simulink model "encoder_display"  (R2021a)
settings: Solver=FixedStepDiscrete  StartTime=0.0  StopTime=Inf  RelTol=1e-3  EnableMultiTasking=on
undefined symbols (not defined in the file or in its folder): Count, edge, falling, resolution, rising, the
libraries: c2806xlib x10, simulink x1, c280xlib x1

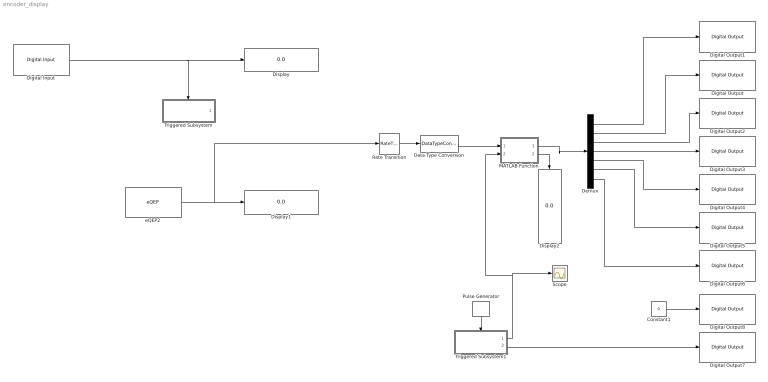
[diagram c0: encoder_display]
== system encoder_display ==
  Constant1 : Constant  Value=0
  Data Type Conversion : DataTypeConversion  OutDataTypeStr=uint16
  Demux : Demux  Outputs=7
  Digital Input : c2806xlib/Digital Input  Commented=on  GPIO_Number=GPIO50~GPIO55  GPIO_Bit0=off  GPIO_Bit1=off  GPIO_Bit2=off  GPIO_Bit3=off  GPIO_Bit4=on  GPIO_Bit5=off  GPIO_Bit6=off  GPIO_Bit7=off  sampleTime=0.1  dataType=auto  GPIO_Bit0_Qualification=Sync to SYSCLKOUT  GPIO_Bit1_Qualification=Sync to SYSCLKOUT  GPIO_Bit2_Qualification=Sync to SYSCLKOUT  GPIO_Bit3_Qualification=Sync to SYSCLKOUT  GPIO_Bit4_Qualification=Sync to SYSCLKOUT  GPIO_Bit5_Qualification=Sync to SYSCLKOUT  GPIO_Bit6_Qualification=Sync to SYSCLKOUT  GPIO_Bit7_Qualification=Sync to SYSCLKOUT  Qualification_Period=-1
  Digital Output : c2806xlib/Digital Output  GPIO_Number=GPIO16~GPIO23  GPIO_Bit0=off  GPIO_BIT0_Toggle=off  GPIO_Bit1=off  GPIO_BIT1_Toggle=off  GPIO_Bit2=off  GPIO_BIT2_Toggle=off  GPIO_Bit3=on  GPIO_BIT3_Toggle=off  GPIO_Bit4=off  GPIO_BIT4_Toggle=off  GPIO_Bit5=off  GPIO_BIT5_Toggle=off  GPIO_Bit6=off  GPIO_BIT6_Toggle=off  GPIO_Bit7=off  GPIO_BIT7_Toggle=off
  Digital Output1 : c2806xlib/Digital Output  GPIO_Number=GPIO50~GPIO55  GPIO_Bit0=off  GPIO_BIT0_Toggle=off  GPIO_Bit1=off  GPIO_BIT1_Toggle=off  GPIO_Bit2=on  GPIO_BIT2_Toggle=off  GPIO_Bit3=off  GPIO_BIT3_Toggle=off  GPIO_Bit4=off  GPIO_BIT4_Toggle=off  GPIO_Bit5=off  GPIO_BIT5_Toggle=off  GPIO_Bit6=off  GPIO_BIT6_Toggle=off  GPIO_Bit7=off  GPIO_BIT7_Toggle=off
  Digital Output2 : c2806xlib/Digital Output  GPIO_Number=GPIO8~GPIO15  GPIO_Bit0=off  GPIO_BIT0_Toggle=off  GPIO_Bit1=off  GPIO_BIT1_Toggle=off  GPIO_Bit2=off  GPIO_BIT2_Toggle=off  GPIO_Bit3=off  GPIO_BIT3_Toggle=off  GPIO_Bit4=off  GPIO_BIT4_Toggle=off  GPIO_Bit5=on  GPIO_BIT5_Toggle=off  GPIO_Bit6=off  GPIO_BIT6_Toggle=off  GPIO_Bit7=off  GPIO_BIT7_Toggle=off
  Digital Output3 : c2806xlib/Digital Output  GPIO_Number=GPIO0~GPIO7  GPIO_Bit0=off  GPIO_BIT0_Toggle=off  GPIO_Bit1=off  GPIO_BIT1_Toggle=off  GPIO_Bit2=off  GPIO_BIT2_Toggle=off  GPIO_Bit3=off  GPIO_BIT3_Toggle=off  GPIO_Bit4=off  GPIO_BIT4_Toggle=off  GPIO_Bit5=on  GPIO_BIT5_Toggle=off  GPIO_Bit6=off  GPIO_BIT6_Toggle=off  GPIO_Bit7=off  GPIO_BIT7_Toggle=off
  Digital Output4 : c2806xlib/Digital Output  GPIO_Number=GPIO16~GPIO23  GPIO_Bit0=off  GPIO_BIT0_Toggle=off  GPIO_Bit1=on  GPIO_BIT1_Toggle=off  GPIO_Bit2=off  GPIO_BIT2_Toggle=off  GPIO_Bit3=off  GPIO_BIT3_Toggle=off  GPIO_Bit4=off  GPIO_BIT4_Toggle=off  GPIO_Bit5=off  GPIO_BIT5_Toggle=off  GPIO_Bit6=off  GPIO_BIT6_Toggle=off  GPIO_Bit7=off  GPIO_BIT7_Toggle=off
  Digital Output5 : c2806xlib/Digital Output  GPIO_Number=GPIO0~GPIO7  GPIO_Bit0=off  GPIO_BIT0_Toggle=off  GPIO_Bit1=off  GPIO_BIT1_Toggle=off  GPIO_Bit2=off  GPIO_BIT2_Toggle=off  GPIO_Bit3=off  GPIO_BIT3_Toggle=off  GPIO_Bit4=on  GPIO_BIT4_Toggle=off  GPIO_Bit5=off  GPIO_BIT5_Toggle=off  GPIO_Bit6=off  GPIO_BIT6_Toggle=off  GPIO_Bit7=off  GPIO_BIT7_Toggle=off
  Digital Output6 : c2806xlib/Digital Output  GPIO_Number=GPIO40~GPIO44  GPIO_Bit0=off  GPIO_BIT0_Toggle=off  GPIO_Bit1=off  GPIO_BIT1_Toggle=off  GPIO_Bit2=off  GPIO_BIT2_Toggle=off  GPIO_Bit3=off  GPIO_BIT3_Toggle=off  GPIO_Bit4=on  GPIO_BIT4_Toggle=off  GPIO_Bit5=off  GPIO_BIT5_Toggle=off  GPIO_Bit6=off  GPIO_BIT6_Toggle=off  GPIO_Bit7=off  GPIO_BIT7_Toggle=off
  Digital Output7 : c2806xlib/Digital Output  GPIO_Number=GPIO0~GPIO7  GPIO_Bit0=on  GPIO_BIT0_Toggle=off  GPIO_Bit1=on  GPIO_BIT1_Toggle=off  GPIO_Bit2=on  GPIO_BIT2_Toggle=off  GPIO_Bit3=on  GPIO_BIT3_Toggle=off  GPIO_Bit4=off  GPIO_BIT4_Toggle=off  GPIO_Bit5=off  GPIO_BIT5_Toggle=off  GPIO_Bit6=off  GPIO_BIT6_Toggle=off  GPIO_Bit7=off  GPIO_BIT7_Toggle=off
  Digital Output8 : c2806xlib/Digital Output  GPIO_Number=GPIO16~GPIO23  GPIO_Bit0=on  GPIO_BIT0_Toggle=off  GPIO_Bit1=off  GPIO_BIT1_Toggle=off  GPIO_Bit2=off  GPIO_BIT2_Toggle=off  GPIO_Bit3=off  GPIO_BIT3_Toggle=off  GPIO_Bit4=off  GPIO_BIT4_Toggle=off  GPIO_Bit5=off  GPIO_BIT5_Toggle=off  GPIO_Bit6=off  GPIO_BIT6_Toggle=off  GPIO_Bit7=off  GPIO_BIT7_Toggle=off
  Display : Display
  Display1 : Display
  Display2 : Display
  MATLAB Function : MATLAB Function  TreatAsAtomicUnit=on
  Pulse Generator : DiscretePulseGenerator  SampleTime=0.0005
  Rate Transition : RateTransition
  Scope : Scope
  Triggered Subsystem : Subsystem  Commented=on  TreatAsAtomicUnit=on
  Triggered Subsystem1 : Subsystem  TreatAsAtomicUnit=on
  eQEP2 : c280xlib/eQEP  useModule=eQEP2  pcInputmode=Quadrature-count  externalClockrate=2x resolution: Count the rising/falling edge  swapPolarityselection=Clockwise  qdfOutputport=off  qapPolarityselection=off  qbpPolarityselection=off  qipPolarityselection=off  qspPolarityselection=off  igatePolarityselection=off  sampleTime=0.01  pcOutputport=on  pcMaximumvalue=999  indexInitializationcheck=off  indexInitializationevent=Rising edge  strobeInitializationcheck=off  strobeInitializationevent=Rising edge  softwareInitializationcheck=on  softwareInitializationsource=Set to init value at start up  softwareInitializationmode=on  pcInitialvalue=0  pcResetmode=Reset on an index event  ieloutputport=off  indexEventlatch=Rising edge  seloutputport=off  strobeEventlatch=Rising edge  pcefOutputport=off  enableEqepcapture=off  qctmrOutputport=off  qcprdOutputport=off  captureTimerprescaler=128  upEventprescaler=128  overflowErrorflag=off  directionErrorflag=off  captureTimerposition=On position counter read  unitTimerperiod=100000000  captureTimerlatch=off  capturePeriodlatch=off  positionCounterlatch=off  soenPolarityselection=off  spselPolarityselection=Index pin is used for sync output  compareValuesource=Specify via dialog  shadowMode=Load on QPOSCNT=0  compareValue=4294967295  syncOutputwidth=1  polaritySyncoutput=Active high  watchdogEnable=off  watchdogTimer=65535  outport1Datatype=auto  outport2Datatype=auto  outport3Datatype=auto  outport4Datatype=auto  outport5Datatype=auto  outport6Datatype=auto  outport7Datatype=auto  outport8Datatype=auto  outport9Datatype=auto  outport10Datatype=auto  outport11Datatype=auto  outport12Datatype=auto  eqepinterrupt_pce=off  eqepinterrupt_qpe=off  eqepinterrupt_qdc=off  eqepinterrupt_wto=off  eqepinterrupt_pcu=off  eqepinterrupt_pco=off  eqepinterrupt_pcr=off  eqepinterrupt_pcm=off  eqepinterrupt_sel=off  eqepinterrupt_iel=off  eqepinterrupt_uto=off  pheOutputport=off  watchdogOutputport=off  outport13Datatype=auto  outport14Datatype=auto
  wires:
  Digital Input/1 -> Triggered Subsystem/Trigger, Display/1
  eQEP2/1 -> Display1/1, Rate Transition/1
  Demux/1 -> Digital Output1/1
  Demux/2 -> Digital Output/1
  Demux/3 -> Digital Output2/1
  Demux/4 -> Digital Output3/1
  Demux/5 -> Digital Output4/1
  Demux/6 -> Digital Output5/1
  Demux/7 -> Digital Output6/1
  MATLAB Function/1(y) -> Demux/1
  Constant1/1 -> Digital Output8/1
  Pulse Generator/1 -> Triggered Subsystem1/Trigger
  Triggered Subsystem1/2(digit) -> Digital Output7/1
  Triggered Subsystem1/1(n) -> Scope/1, MATLAB Function/2(digit)
  Rate Transition/1 -> Data Type Conversion/1
  Data Type Conversion/1 -> MATLAB Function/1(num)
  MATLAB Function/2(w) -> Display2/1

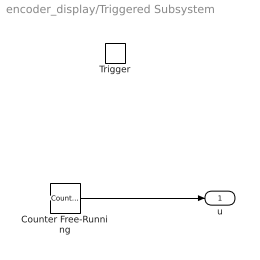
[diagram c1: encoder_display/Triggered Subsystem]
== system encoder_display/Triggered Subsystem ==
  Trigger : TriggerPort  VariantControl=(inherit)
  Counter Free-Running : simulink/Sources/Counter Free-Running  NumBits=12  tsamp=-1
  u : Outport
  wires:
  Counter Free-Running/1 -> u/1

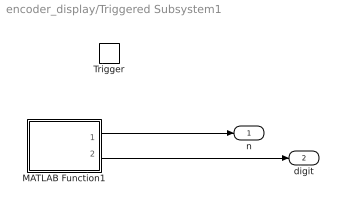
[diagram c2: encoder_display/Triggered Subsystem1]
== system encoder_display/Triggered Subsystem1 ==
  Trigger : TriggerPort  VariantControl=(inherit)
  MATLAB Function1 : MATLAB Function  TreatAsAtomicUnit=on
  n : Outport
  digit : Outport  Port=2
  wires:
  MATLAB Function1/1(nn) -> n/1
  MATLAB Function1/2(digit) -> digit/1

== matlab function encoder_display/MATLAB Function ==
function [y,w]= fcn(num,digit)

  segments = [0 0 0 0 0 0 0]
  x = uint16(0)
  

    
    k   = idivide(num,1000);
    num = num - k*1000;
        
    h  = idivide(num,100);
    num = num - h*100;
        
    da = idivide( num,10 );
    num = num - da*10;
      
    u  = num;
        
        
    switch digit 
        case 0
            % u
            x = u;
        case 1
            % da
            x = da;
        case 2
            % h
            x = h;
        case 3
            % k
            x = k;
            
    end
        
    
switch x
    case 0
        segments = [1 1 1 1 1 1 0]
    case 1
        segments = [0 1 1 0 0 0 0]
    case 2
        segments = [1 1 0 1 1 0 1]
    case 3
        segments = [1 1 1 1 0 0 1]
    case 4
        segments = [0 1 1 0 0 1 1]
    case 5
        segments = [1 0 1 1 0 1 1]
    case 6
        segments = [1 0 1 1 1 1 1]
    case 7
        segments = [1 1 1 0 0 0 0]
    case 8
        segments = [1 1 1 1 1 1 1]
    case 9
        segments = [1 1 1 0 0 1 1]
    otherwise
        segments = [0 0 0 0 0 0 1]

end


y = segments
w = [k h da u];

== matlab function encoder_display/Triggered
Subsystem1/MATLAB Function1 ==
function [nn, digit]= fcn


    persistent n

    digit = [1 0 0 0]
        
    if isempty(n)
        n = 0;
    else
        n = n+1;
    end
    
    if n>3
        n=0;
    end
  
    switch n
        case 3
            digit = [0 0 0 1]
        case 2
            digit = [0 0 1 0]
        case 1
            digit = [0 1 0 0]
        case 0
            digit = [1 0 0 0]
    end
    nn=n

y = [nn,digit];
